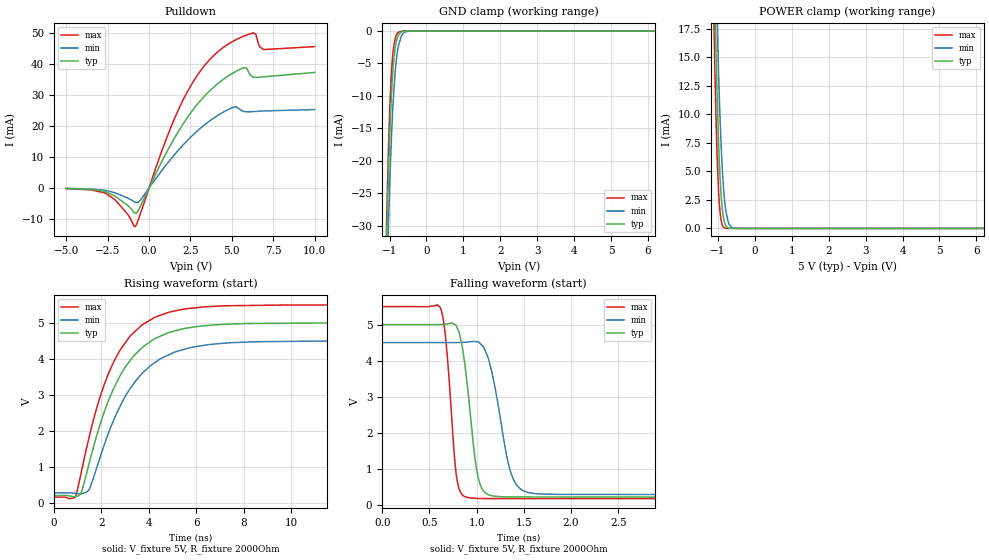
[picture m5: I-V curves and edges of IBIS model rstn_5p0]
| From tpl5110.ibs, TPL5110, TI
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|   Model
[Model]   rstn_5p0
Model_type   I/O_open_drain
Polarity   Non-Inverting
Enable   Active-Low
Vinl = 1.5
Vinh = 3.5
Vmeas = 2.5
Vref = 5
Cref = 1pF
Rref = 2000
|   typ   min   max
C_comp   0.474pF   0.343pF   0.582pF
[Voltage Range]   5   4.5   5.5
[Temperature Range]   25   105   -40
[Pullup Reference]   5   4.5   5.5
[Pulldown Reference]   0   0   0
[Power Clamp Reference]   5   4.5   5.5
[GND Clamp Reference]   0   0   0
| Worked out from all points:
|   slope of the pulldown table from 0 to 0.75 V, typ, clamps not added: 90.8 ohm
|   GND clamp passes 1 mA (typ) near -0.78 V on its own axis
|   POWER clamp passes 1 mA (typ) near -0.85 V on its own axis
|   falling waveform, V_fixture 5V, R_fixture 2000Ohm: 20-80 % time 121ps typ, 174ps min, 90.1ps max; typ from 5 V to 0.212 V
|   rising waveform, V_fixture 5V, R_fixture 2000Ohm: 20-80 % time 1.8ns typ, 1.93ns min, 1.71ns max; typ from 0.212 V to 5 V
[Pulldown]
|   Voltage   I(typ)   I(min)   I(max)
-5V       -132.5uA   -121.1uA   -187.6uA
-2.615V   -1.207mA   -775.6uA   -1.727mA
-845mV    -8.114mA   -4.573mA   -12.43mA
-545mV    -6.147mA   -4.034mA   -8.648mA
1.69V     17.46mA    11.68mA    24.19mA
2.74V     25.75mA    17.51mA    34.85mA
3.82V     32.07mA    22.2mA     42.2mA
5.185V    37.36mA    26.14mA    47.58mA
5.695V    38.72mA    24.67mA    48.84mA
6.31V     35.7mA     24.61mA    49.98mA
6.925V    35.82mA    24.81mA    44.59mA
10V       37.21mA    25.26mA    45.53mA
[GND Clamp]
|   Voltage   I(typ)   I(min)   I(max)
-5V       -1.486A    -1.386A    -1.583A
-1.085V   -33.82mA   -41.23mA   -30.54mA
-1.07V    -30.36mA   -37.93mA   -26.82mA
-1.04V    -23.96mA   -31.7mA    -20.08mA
-995mV    -15.88mA   -23.39mA   -12mA
-950mV    -9.811mA   -16.49mA   -6.492mA
-905mV    -5.688mA   -11.08mA   -3.207mA
-845mV    -2.519mA   -6.091mA   -1.09mA
-755mV    -568.8uA   -2.164mA   -172.6uA
-620mV    -28.9uA    -276.8uA   -5.951uA
-440mV    -185.4nA   -4.113uA   -392.6nA
10V       0A         0A         0A
[POWER Clamp]
|   Voltage   I(typ)   I(min)   I(max)
-5V       994.4mA    930mA      1.055A
-1.115V   24.99mA    31.72mA    19.12mA
-1.1V     22.53mA    29.35mA    16.61mA
-1.07V    17.92mA    24.82mA    12.05mA
-1.01V    10.22mA    16.76mA    5.231mA
-980mV    7.254mA    13.32mA    3.075mA
-905mV    2.505mA    6.675mA    552uA
-860mV    1.136mA    4.046mA    140.6uA
-815mV    450.8uA    2.293mA    26.37uA
-695mV    16.42uA    347.8uA    106.1nA
-485mV    430.8nA    2.287uA    0A
10V       0A         0A         0A
[Ramp]
R_load = 2000
|   typ   min   max
dV/dt_r   2.87295/1.79792e-09   2.5299/1.93113e-09   3.19996/1.71215e-09
dV/dt_f   2.87295/1.21092e-10   2.5299/1.73517e-10   3.19996/9.01041e-11
[Falling Waveform]
V_fixture = 5V
V_fixture_min = 4.5V
V_fixture_max = 5.5V
R_fixture = 2000Ohm
C_fixture = 0F
|   Time   V(typ)   V(min)   V(max)
0s        5V         4.5V       5.5V
618ps     5.003V     4.5V       5.466V
667.4ps   5.011V     4.5V       4.741V
795.8ps   4.896V     4.5V       640mV
872.3ps   3.955V     4.51V      229.2mV
1ns       969.7mV    4.524V     174.3mV
1.123ns   281mV      4.071V     170.8mV
1.39ns    216.9mV    700.7mV    168.3mV
1.733ns   213.8mV    292.5mV    166.8mV
50ns      211.8mV    283.5mV    166.7mV
[Rising Waveform]
V_fixture = 5V
V_fixture_min = 4.5V
V_fixture_max = 5.5V
R_fixture = 2000Ohm
C_fixture = 0F
|   Time   V(typ)   V(min)   V(max)
0s        211.8mV    283.5mV    166.7mV
934.4ps   187.3mV    270.8mV    227.4mV
1.143ns   279.9mV    257mV      820mV
1.497ns   1.128V     394.9mV    1.861V
2.109ns   2.505V     1.593V     3.264V
2.783ns   3.529V     2.682V     4.242V
4.078ns   4.489V     3.822V     5.089V
5.512ns   4.848V     4.273V     5.389V
11.25ns   4.999V     4.498V     5.498V
50ns      5V         4.5V       5.5V
